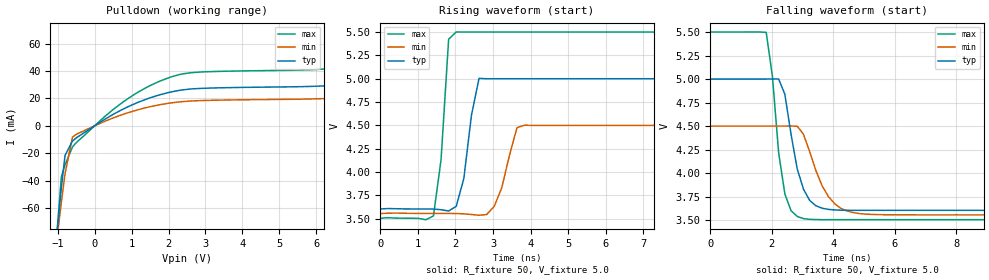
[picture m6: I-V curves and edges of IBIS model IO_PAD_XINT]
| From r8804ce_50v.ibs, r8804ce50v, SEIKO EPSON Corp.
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[Model]   IO_PAD_XINT
Model_type Open_drain
Enable Active-High
Polarity Non-Inverting
Vref=5.5
Vmeas=2.50
Rref=5000
C_comp   2.5p   2.0p   3.0p
[Temperature Range] 25   105   -40
[Voltage Range]   5.0   4.5   5.5
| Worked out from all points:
|   slope of the pulldown table from 0 to 0.75 V, typ, clamps not added: 63 ohm
|   falling waveform, R_fixture 50, V_fixture 5.0: 20-80 % time 499ps typ, 717ps min, 378ps max; typ from 5 V to 3.6 V
|   rising waveform, R_fixture 50, V_fixture 5.0: 20-80 % time 292ps typ, 381ps min, 228ps max; typ from 3.6 V to 5 V
[Pulldown]
-5V       -1.358A    -1.099A    -1.697A
-1.1V     -101.8mA   -101.1mA   -106mA
-900mV    -45.15mA   -55.82mA   -37.2mA
-800mV    -21.58mA   -34.92mA   -28.5mA
-600mV    -11.21mA   -8.18mA    -15.49mA
800mV     12.6mA     8.658mA    18mA
2V        24.33mA    16.48mA    35.1mA
2.7V      27.11mA    18.26mA    39.04mA
7.3V      32.25mA    22.11mA    45.83mA
8.3V      39mA       26.99mA    55.11mA
9.4V      51.58mA    36.18mA    72.08mA
10V       60.61mA    42.84mA    84.12mA
[Falling Waveform]
R_fixture=50
V_fixture=5.0
V_fixture_min=4.5
V_fixture_max=5.5
0s        5V         4.5V       5.5V
1.818ns   5V         4.5V       5.496V
2.02ns    5V         4.5V       5.026V
2.222ns   5.001V     4.5V       4.217V
2.424ns   4.838V     4.5V       3.779V
2.828ns   4.042V     4.498V     3.54V
3.03ns    3.829V     4.413V     3.517V
3.838ns   3.615V     3.753V     3.506V
4.848ns   3.605V     3.571V     3.506V
20ns      3.605V     3.557V     3.506V
[Rising Waveform]
R_fixture=50
V_fixture=5.0
V_fixture_min=4.5
V_fixture_max=5.5
0s        3.605V     3.557V     3.506V
1.414ns   3.604V     3.557V     3.53V
1.616ns   3.597V     3.557V     4.132V
1.818ns   3.584V     3.557V     5.423V
2.02ns    3.634V     3.556V     5.501V
2.626ns   5.004V     3.538V     5.5V
3.03ns    5V         3.633V     5.5V
3.636ns   5V         4.476V     5.5V
3.838ns   5V         4.502V     5.5V
20ns      5V         4.5V       5.5V
[Ramp]
R_load=50
dV/dt_r   8.371E-1/2.509E-10   5.659E-1/3.448E-10   1.197E+0/1.926E-10
dV/dt_f   8.371E-1/4.844E-10   5.659E-1/7.069E-10   1.197E+0/3.438E-10
|[End   IO_PAD_XINT
